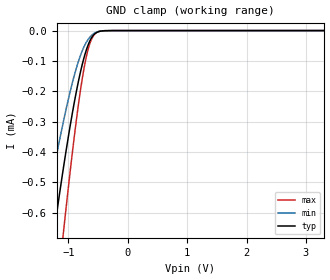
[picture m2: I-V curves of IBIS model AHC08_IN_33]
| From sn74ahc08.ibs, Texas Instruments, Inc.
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[Model]   AHC08_IN_33
Model_type  Input
Vinl=0.9
Vinh=2.34
| variable   typ   min   max
C_comp   0.84pF   0.74pF   0.96pF
[Temperature Range]   40   100   -40
| Ambient temperature   25   85   -40
[Voltage range]   3.3   3   3.6
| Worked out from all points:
|   GND clamp passes 1 mA (typ) near -1.47 V on its own axis
[GND Clamp]
| AHC08_IN_33
|   Voltage   I(typ)   I(min)   I(max)
-5.5V     -8.894mA   -6.578mA   -10.58mA
-1.455V   -977uA     -680.1uA   -1.39mA
-1.425V   -931.5uA   -646.9uA   -1.329mA
-1.235V   -654.9uA   -445.9uA   -951.4uA
-1.08V    -447.6uA   -296.2uA   -658.7uA
-900mV    -236.1uA   -147.3uA   -348.2uA
-765mV    -110.3uA   -65.75uA   -156.6uA
-710mV    -71.34uA   -42.68uA   -97.12uA
-645mV    -36.78uA   -23.24uA   -46.24uA
-535mV    -7.694uA   -5.88uA    -7.629uA
-250mV    -25.43nA   -25nA      -9.199nA
3.3V      1.095nA    186.2pA    5.229nA
